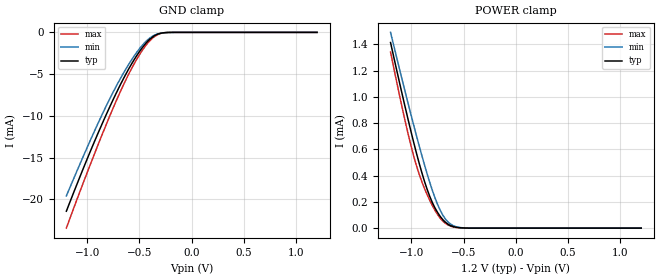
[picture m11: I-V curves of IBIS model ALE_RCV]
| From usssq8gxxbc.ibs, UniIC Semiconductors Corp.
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|   Model ALE_RCV
[Model] ALE_RCV
Model_type Input
Polarity   Non-Inverting
Enable   Active-High
Vinl =  2.400E-01
Vinh =  9.600E-01
C_comp   3.805E-13   3.618E-13   4.037E-13
C_comp_power_clamp   1.480E-13   1.410E-13   1.552E-13
C_comp_gnd_clamp   2.042E-13   1.927E-13   2.415E-13
[Model Spec]
Vinh   9.600E-01   9.120E-01   1.008E+00
Vinl   2.400E-01   2.280E-01   2.520E-01
[Temperature Range]   4.500E+01   9.500E+01   0.000E+00
[Voltage Range]   1.200E+00   1.140E+00   1.260E+00
[C Comp Corner]
C_comp_power_clamp   1.552E-13   1.480E-13   1.410E-13
C_comp_gnd_clamp   2.042E-13   1.927E-13   2.415E-13
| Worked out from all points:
|   GND clamp passes 1 mA (typ) near -0.41 V on its own axis
|   POWER clamp passes 1 mA (typ) near -1.08 V on its own axis
[GND_clamp]
|Voltage   I(typ)   I(min)   I(max)
-1.2V     -21.41mA   -19.58mA   -23.44mA
-1.05V    -16.66mA   -15.19mA   -18.4mA
-900mV    -12.17mA   -10.97mA   -13.57mA
-775mV    -8.663mA   -7.718mA   -9.731mA
-675mV    -6.07mA    -5.357mA   -6.872mA
-575mV    -3.768mA   -3.276mA   -4.32mA
-500mV    -2.298mA   -1.958mA   -2.676mA
-425mV    -1.123mA   -929.9uA   -1.344mA
-375mV    -561.1uA   -457.6uA   -689.4uA
-300mV    -117.3uA   -101.1uA   -143uA
-225mV    -12.89uA   -13.99uA   -12.5uA
1.2V      0A         0A         0A
[POWER_clamp]
|Voltage   I(typ)   I(min)   I(max)
-1.2V     1.414mA    1.491mA    1.341mA
-1.1V     1.059mA    1.166mA    959.1uA
-1.025V   804.3uA    928.4uA    694.9uA
-975mV    642.7uA    774.1uA    539.3uA
-925mV    491.6uA    624.7uA    408.5uA
-850mV    296.4uA    414.1uA    255.5uA
-775mV    154.4uA    231.8uA    135.8uA
-700mV    65.09uA    99.41uA    53.85uA
-625mV    19.16uA    30.35uA    15.25uA
-550mV    3.935uA    6.436uA    3.094uA
-450mV    345.4nA    637.5nA    233.6nA
1.2V      0A         0A         1.66nA
